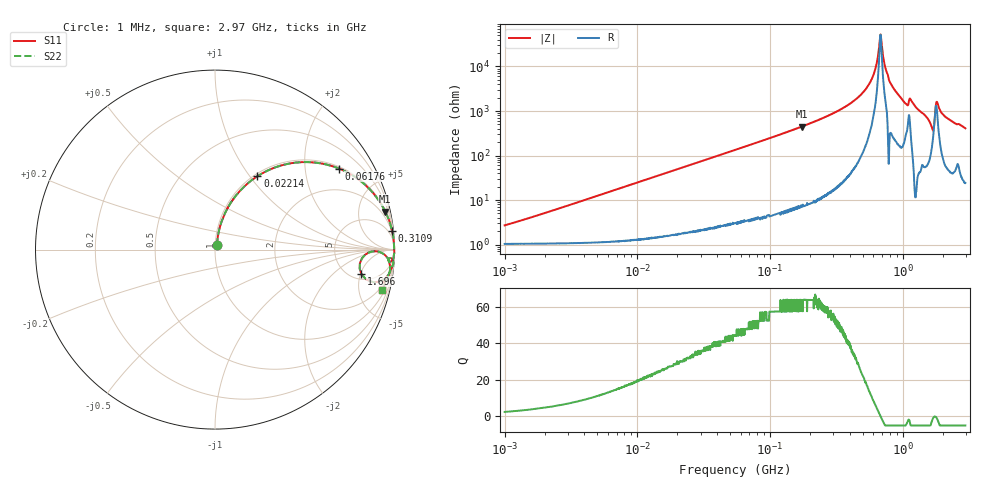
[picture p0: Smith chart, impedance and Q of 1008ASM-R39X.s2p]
!s-Parameter Generated by FASTRON Sdn. Bhd.
!FASTRON P/N : 1008ASM-R39X
!Keysight Technologies: E4991B_MY54100416_A.01.15
!Date: Tue Nov 21 09:15:26 2023
!Version  :Rev00  Wed Nov 22 15:15:09 2023
!Data & Calibration Information:
!Freq  S11  S21  S12  S22
!PortZ  Port1:50+j0  Port2:50+j0
!When reading reference impedance value at option line is always used.
! Remarks : This data is being provided solely for informational purposes.
# Hz S dB R 50
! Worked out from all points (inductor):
!   1599 points, 1 MHz to 2.97 GHz, reference 50 ohm
!   read as one part in series: L = 397 nH near 1.253 MHz
!   highest Q = 63.7 at 173.1 MHz (marker M1), where L = 409 nH
!   self-resonance near 678.7 MHz
!   S11 on the Smith chart (normalised r, x): 1 MHz: 1.02, +0.05; 22.14 MHz: 1.04, +1.09; 61.76 MHz: 1.06, +3.02; 310.9 MHz: 1, +19; 1.696 GHz: 6.11, -5.10; 2.97 GHz: 1.48, -8.12
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1000000  -31.50 66.0  -0.09 -1.4  -0.09 -1.4  -31.50 66.0
3804036  -20.60 78.1  -0.13 -5.3  -0.13 -5.3  -20.60 78.1
1.439846e7  -9.61 68.3  -0.63 -19.3  -0.63 -19.3  -9.61 68.3
2.214172e7  -6.52 60.0  -1.25 -28.1  -1.25 -28.1  -6.52 60.0
5.477226e7  -2.01 36.2  -4.56 -52.5  -4.56 -52.5  -2.01 36.2
6.176144e7  -1.66 33.1  -5.26 -55.7  -5.26 -55.7  -1.66 33.1
1.731398e8  -0.24 12.6  -13.20 -76.5  -13.20 -76.5  -0.24 12.6
2.073156e8  -0.17 10.3  -15.00 -78.8  -15.00 -78.8  -0.17 10.3
3.10929e8  -0.07 6.1  -19.50 -82.8  -19.50 -82.8  -0.07 6.1
4.413523e8  -0.03 3.2  -25.20 -85.0  -25.20 -85.0  -0.03 3.2
5.418594e8  -0.02 1.6  -30.90 -84.9  -30.90 -84.9  -0.02 1.6
6.140682e8  -0.02 0.7  -37.70 -81.2  -37.70 -81.2  -0.02 0.7
6.787043e8  -0.02 0.0  -54.20 -12.0  -54.20 -12.0  -0.02 0.0
6.958997e8  -0.02 -0.2  -49.60 55.3  -49.60 55.3  -0.02 -0.2
7.846996e8  -0.00 -1.1  -34.40 88.2  -34.40 88.2  -0.00 -1.1
1.0437e9  -0.11 -3.7  -23.60 76.8  -23.60 76.8  -0.11 -3.7
1.159346e9  -0.08 -3.3  -24.80 79.4  -24.80 79.4  -0.08 -3.3
1.534307e9  -0.20 -8.1  -17.00 76.9  -17.00 76.9  -0.20 -8.1
1.695807e9  -1.67 -9.3  -12.80 35.7  -12.80 35.7  -1.67 -9.3
1.827992e9  -0.30 -3.1  -24.00 56.6  -24.00 56.6  -0.30 -3.1
2.124078e9  -0.17 -7.8  -17.30 77.8  -17.30 77.8  -0.17 -7.8
2.970126e9  -0.37 -13.6  -12.60 73.0  -12.60 73.0  -0.37 -13.6
